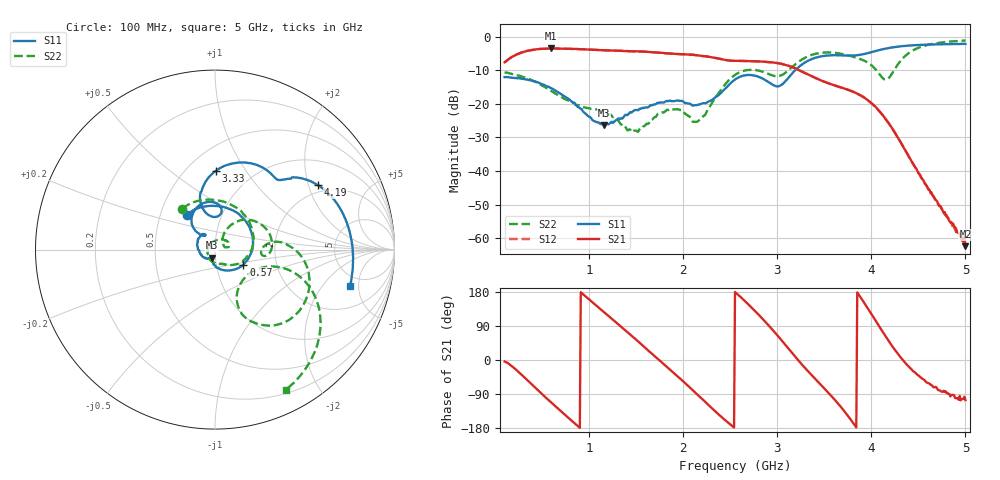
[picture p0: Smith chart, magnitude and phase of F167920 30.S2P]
!  2-Port S-parameters saved by WinCal
! VAR MeasName=S-Parameters (CALIBRATED_DATA) read from VNA (N5242A)
! VAR MeasDate=2016-11-22 9:56:38
! VAR NAME=F167920 30
! VAR FILENAME=F167920 30.S2P
! VAR DATE=2016-11-22 9:56:38
! VAR PHYS_PORTS=1,2
# Hz S DB R 50
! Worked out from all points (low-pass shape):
!   491 points, 100 MHz to 5 GHz, reference 50 ohm
!   highest |S21| = -3.53 dB at 590 MHz (marker M1); lowest = -62.3 dB at 5 GHz (marker M2)
!   |S21| within 3 dB of the highest: 152 MHz to 2.376 GHz (2.224 GHz wide, 176 % of centre)
!   lowest |S11| = -26.3 dB at 1.16 GHz (marker M3), VSWR 1.10, Z = 48.3 - j4.44 ohm
!   |S11| at or under -10 dB: start of sweep to 3.189 GHz
!   |S22| runs from -28.4 to -1.2 dB; largest |S21 - S12| = 0.0011
!   S11 on the Smith chart (normalised r, x): 100 MHz: 0.68, +0.28; 570 MHz: 1.35, -0.24; 3.33 GHz: 0.68, +0.74; 4.19 GHz: 1.75, +2.32; 5 GHz: 3.87, -3.97
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1e8  -12.07 128.7  -7.65 -3.9  -7.64 -3.9  -10.70 128.4
3e8  -12.61 46.7  -4.58 -43.3  -4.58 -43.4  -12.04 45.3
5.7e8  -14.91 -27.9  -3.57 -106.2  -3.58 -106.2  -15.54 -24.1
5.9e8  -15.25 -33.6  -3.53 -110.9  -3.54 -111.0  -16.05 -28.4
7.6e8  -18.20 -67.8  -3.63 -148.7  -3.63 -148.7  -18.80 -48.6
9.2e8  -21.57 -95.4  -3.74 176.8  -3.74 176.8  -20.80 -62.4
1.16e9  -26.29 -108.9  -4.07 125.5  -4.07 125.5  -22.45 -88.7
1.42e9  -23.00 -137.8  -4.36 70.4  -4.36 70.3  -27.71 -171.6
1.74e9  -19.72 162.7  -4.79 0.6  -4.79 0.6  -22.87 53.2
1.96e9  -19.14 131.7  -5.22 -47.6  -5.22 -47.7  -21.78 17.2
2.12e9  -20.40 125.9  -5.49 -84.4  -5.49 -84.4  -25.35 24.1
2.34e9  -18.09 135.1  -6.35 -135.6  -6.35 -135.6  -18.17 60.0
2.55e9  -12.79 123.4  -7.21 179.6  -7.22 179.5  -11.40 36.6
2.92e9  -13.80 80.6  -7.59 87.9  -7.60 87.9  -11.27 -7.3
3.13e9  -11.86 107.1  -8.79 26.7  -8.80 26.7  -9.75 7.4
3.33e9  -7.14 89.4  -11.32 -30.6  -11.34 -30.7  -5.83 -8.8
3.37e9  -6.64 84.4  -11.85 -41.2  -11.86 -41.3  -5.41 -13.6
3.77e9  -5.66 49.5  -16.00 -153.7  -16.02 -153.7  -5.70 -54.8
4.05e9  -4.24 40.7  -21.06 102.0  -21.12 102.2  -9.90 -67.3
4.19e9  -3.38 31.9  -25.97 47.8  -26.02 48.1  -12.18 -28.9
4.5e9  -2.50 11.4  -40.55 -40.9  -40.57 -40.5  -3.35 -30.9
5e9  -2.16 -14.9  -62.34 -106.0  -61.58 -107.5  -1.16 -63.2
